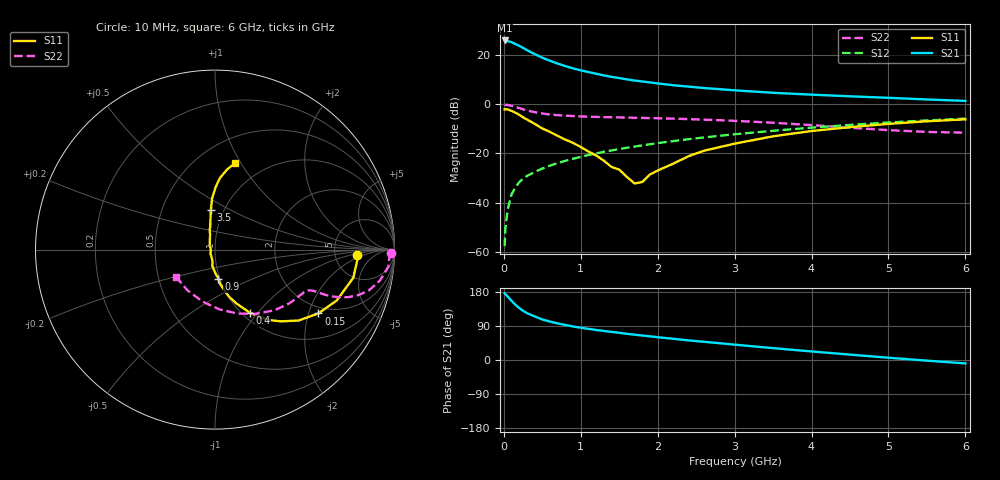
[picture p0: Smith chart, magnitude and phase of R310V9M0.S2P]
! SIEMENS Small Signal Semiconductors
! BFR181
! Si NPN RF Bipolar Junction Transistor in SOT23
! VCE = 10 V  IC = 9 mA
! Common Emitter S-Parameters:  May  1996
# GHz  S  MA  R  50
!  f  S11  S21  S12  S22
! GHz  MAG  ANG  MAG  ANG  MAG  ANG  MAG  ANG
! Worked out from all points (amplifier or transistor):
!   36 points, 10 MHz to 6 GHz, reference 50 ohm
!   highest |S21| = 26.0 dB at 10 MHz (marker M1)
!   |S21| within 3 dB of that: start of sweep to 249 MHz
!   unconditionally stable (mu >= 1): 940.6 MHz to 2.942 GHz
!   at 250 MHz: K = 0.56, MSG = 26.6 dB, |S12| = -30.3 dB
!   at 1.4 GHz: K = 1.04, MAG = 13.7 dB, |S12| = -18.8 dB
!   at 6 GHz: K = 0.87, MSG = 3.6 dB, |S12| = -5.8 dB
!   S11 on the Smith chart (normalised r, x): 10 MHz: 8.38, -1.43; 150 MHz: 1.77, -2.32; 400 MHz: 1.08, -0.91; 900 MHz: 0.98, -0.33; 3.5 GHz: 0.87, +0.41; 6 GHz: 0.74, +0.94
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0.01  0.7923 -2.3  19.91 176.1  0.0013 80.9  0.9823 -1.0
0.02  0.7946 -4.4  19.48 173.9  0.0029 82.1  0.9728 -2.2
0.05  0.7864 -11.5  19.23 167.4  0.0073 84.1  0.9705 -5.7
0.1  0.7351 -22.7  18.4 156.4  0.0147 79.2  0.934 -10.7
0.15  0.6767 -31.7  16.87 145.7  0.0205 73.7  0.8868 -14.9
0.2  0.6109 -40.3  15.52 137.2  0.0261 71.5  0.8381 -17.6
0.25  0.5439 -47.3  14.07 129.7  0.0307 69.0  0.7894 -19.6
0.3  0.4911 -53.0  12.67 123.8  0.0348 69.1  0.7505 -20.8
0.4  0.4019 -61.1  10.54 115.0  0.0421 67.6  0.6929 -22.0
0.5  0.3221 -68.4  8.864 107.0  0.0493 67.9  0.6501 -22.4
0.6  0.274 -73.4  7.683 101.3  0.0567 67.9  0.6209 -22.5
0.7  0.2273 -77.5  6.746 96.6  0.0637 68.4  0.6011 -22.7
0.9  0.1644 -83.2  5.379 88.5  0.0782 68.5  0.5767 -23.2
1.1  0.1094 -93.8  4.527 82.2  0.0929 68.6  0.5603 -24.3
1.4  0.0531 -108.8  3.622 74.1  0.1152 67.9  0.5453 -26.7
1.7  0.0245 -165.0  3.047 66.8  0.1381 66.6  0.5321 -29.6
2.2  0.0618 117.6  2.449 56.0  0.1787 63.8  0.5109 -35.8
2.6  0.1133 105.1  2.145 48.1  0.2114 60.8  0.4872 -41.5
3.5  0.2234 96.0  1.716 31.3  0.2894 53.2  0.4217 -58.1
4.5  0.3431 89.7  1.454 14.2  0.3813 42.8  0.3335 -85.9
5.5  0.4518 81.4  1.255 -1.7  0.4699 30.7  0.2739 -123.9
6  0.4945 77.0  1.173 -9.0  0.5112 24.0  0.2654 -145.6
